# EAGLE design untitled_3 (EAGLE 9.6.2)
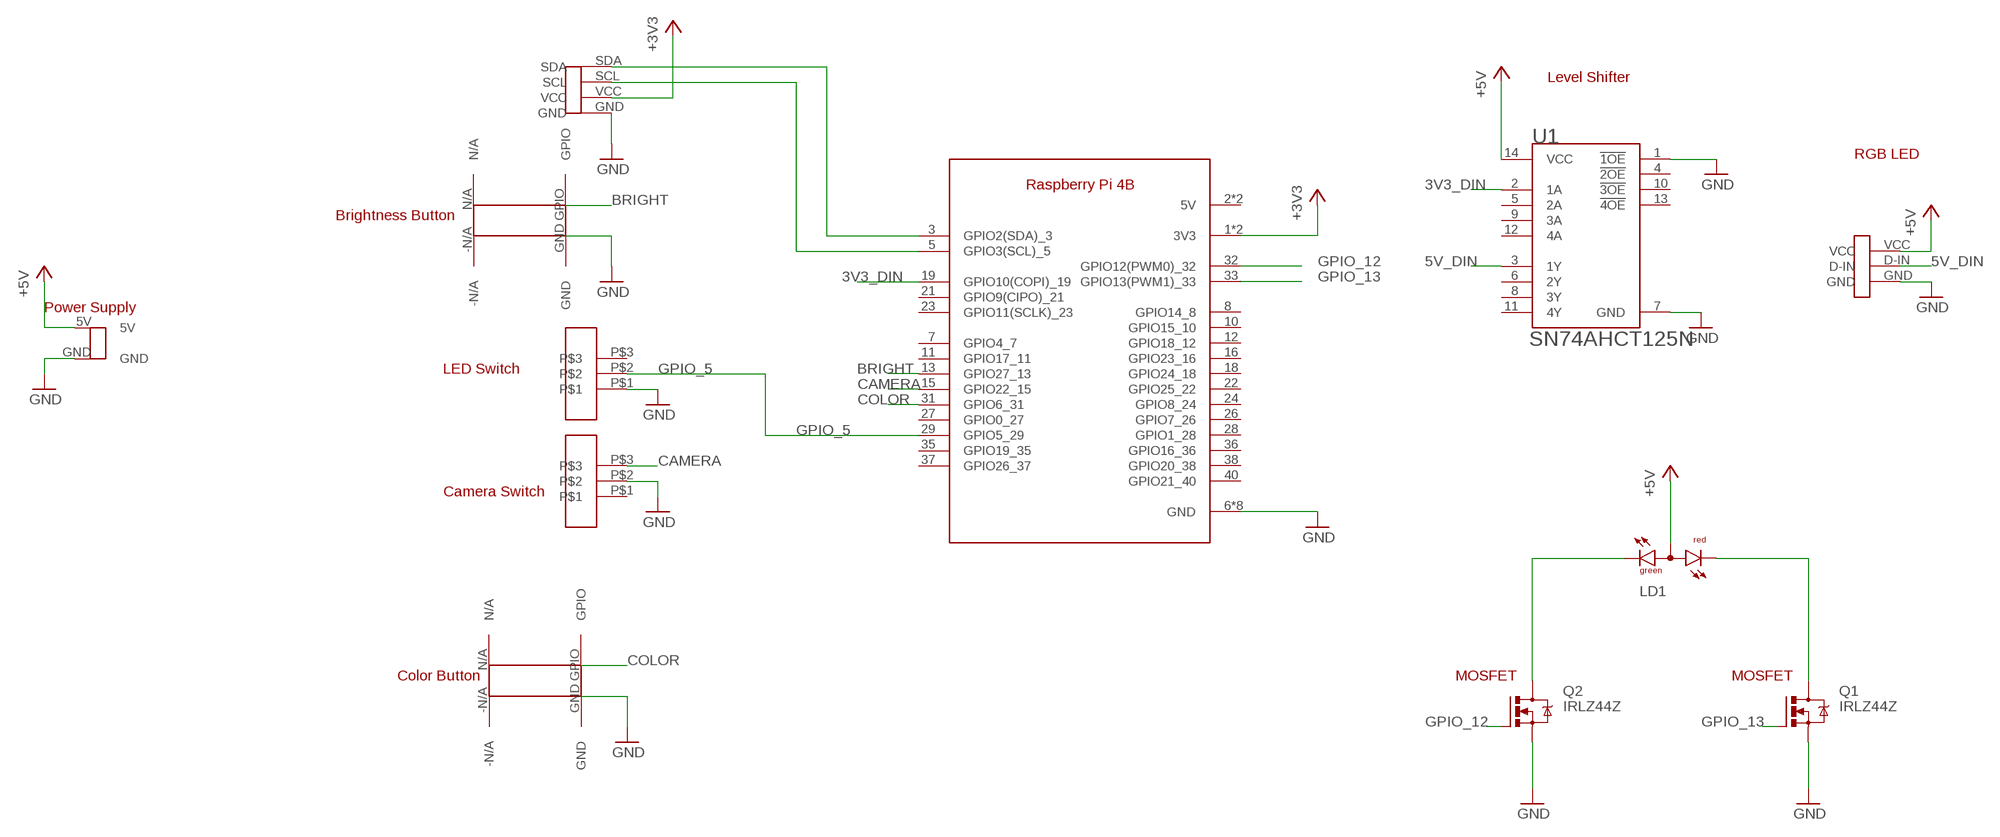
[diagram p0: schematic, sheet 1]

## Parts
LD1  DUOLED-RG-A  [DUOLED-A-5MM]
Q1  IRLZ44Z  [TO220BH]
Q2  IRLZ44Z  [TO220BH]
U1  TEXAS_INSTRUMENTS_SN74AHCT125NTEXAS_INSTRUMENTS_SN74AHCT125N_0_0  [TEXAS_INSTRUMENTS_SN74AHCT125N_0]
U$1  RASPBERRY_PI_4  [RASPI_4B]
U$2  G13-SW  [G13-SW]
U$3  G13-SW  [G13-SW]
U$4  LIGHTSENSOR-PO  [LIGHTSENSOR-IO]
U$5  LED-STRIP-PO  [LED-STRIP-PO]
U$6  G13-BUTTON  [G13-BUTTON]
U$7  G13-BUTTON  [G13-BUTTON]
U$8  G13-BATTERY  [G13-BATTERY]

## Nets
3V3_DIN: U1.2(1A) U$1.19(GPIO10(COPI)_19)
5V_DIN: U1.3(1Y) U$5.D-IN
+3V3: U$1.1(3V3) U$1.17(3V3) U$4.VCC
+5V: LD1.A U1.14(VCC) U$5.VCC U$8.5V
BRIGHT: U$1.13(GPIO27_13) U$6.GPIO
CAMERA: U$1.15(GPIO22_15) U$3.P$3
COLOR: U$1.31(GPIO6_31) U$7.GPIO
GND: Q1.S Q2.S U1.1(!1OE!) U1.7(GND) U$1.6(GND) U$1.9(GND) U$1.14(GND) U$1.20(GND) U$1.25(GND) U$1.30(GND) U$1.34(GND) U$1.39(GND) U$2.P$1 U$3.P$2 U$4.GND U$5.GND U$6.GND U$7.GND U$8.GND
GPIO_5: U$1.29(GPIO5_29) U$2.P$2
GPIO_12: Q2.G U$1.32(GPIO12(PWM0)_32)
GPIO_13: Q1.G U$1.33(GPIO13(PWM1)_33)
N$1: U$1.3(GPIO2(SDA)_3) U$4.SDA
N$2: U$1.5(GPIO3(SCL)_5) U$4.SCL
N$3: LD1.CR Q1.D
N$12: LD1.CX(CG) Q2.D
Unconnected: U1.4(!2OE!) U1.5(2A) U1.6(2Y) U1.8(3Y) U1.9(3A) U1.10(!3OE!) U1.11(4Y) U1.12(4A) U1.13(!4OE!) U$1.2(5V) U$1.4(5V) U$1.7(GPIO4_7) U$1.8(GPIO14_8) U$1.10(GPIO15_10) U$1.11(GPIO17_11) U$1.12(GPIO18_12) U$1.16(GPIO23_16) U$1.18(GPIO24_18) U$1.21(GPIO9(CIPO)_21) U$1.22(GPIO25_22) U$1.23(GPIO11(SCLK)_23) U$1.24(GPIO8_24) U$1.26(GPIO7_26) U$1.27(GPIO0_27) U$1.28(GPIO1_28) U$1.35(GPIO19_35) U$1.36(GPIO16_36) U$1.37(GPIO26_37) U$1.38(GPIO20_38) U$1.40(GPIO21_40) U$2.P$3 U$3.P$1 U$6.-N/A U$6.N/A U$7.-N/A U$7.N/A

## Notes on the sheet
- Level Shifter
- RGB LED
- Brightness Button
- Power Supply
- LED Switch
- Camera Switch
- Color Button | MOSFET | MOSFET

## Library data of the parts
LD1 = led:DUOLED-RG-A: DUO LED 2 colors (red/green), 5 mm, round, common Anode www.ligitek.com or other producers.
Q1 Q2 = transistor-power:IRLZ44Z: N-Channel HEXFET® Power MOSFET Logic Level AUTOMOTIVE MOSFET Source: http://www.irf.com/product-info/datasheets/data/irlz44zpbf.pdf
U1 = Texas Instruments - SN74AHCT125N:TEXAS_INSTRUMENTS_SN74AHCT125N: QUADRUPLE BUS BUFFER GATES WITH 3-STATE OUTPUTS; CENTROID_NOT_SPECIFIED: No; DATASHEET: http://www.ti.com/lit/ds/symlink/sn74ahct125.pdf; DIGIKEY_DESCRIPTION: IC BUS BUFFER TRI-ST QD 14DIP; DIGIKEY_PART_NUMBER: 296-4655-5-ND; IPC_LAND_PATTERN_NAME: DIP794W46P254L1930H508Q14; LEAD_FREE: yes; MF: Texas Instruments; MOUSER_PART_NUMBER: 595-SN74AHCT125N; MPN: SN74AHCT125N; PACKAGE: PDIP-14; PREFIX: U; ROHS: yes; TEMPERATURE_RANGE_HIGH: +125°C; TEMPERATURE_RANGE_LOW: -40°C
U$1 = raspberryPi4:RASPBERRY_PI_4
U$2 U$3 = raspberryPi4:G13-SW
U$4 = raspberryPi4:LIGHTSENSOR-PO
U$5 = raspberryPi4:LED-STRIP-PO
U$6 U$7 = sumayyah:G13-BUTTON
U$8 = raspberryPi4:G13-BATTERY

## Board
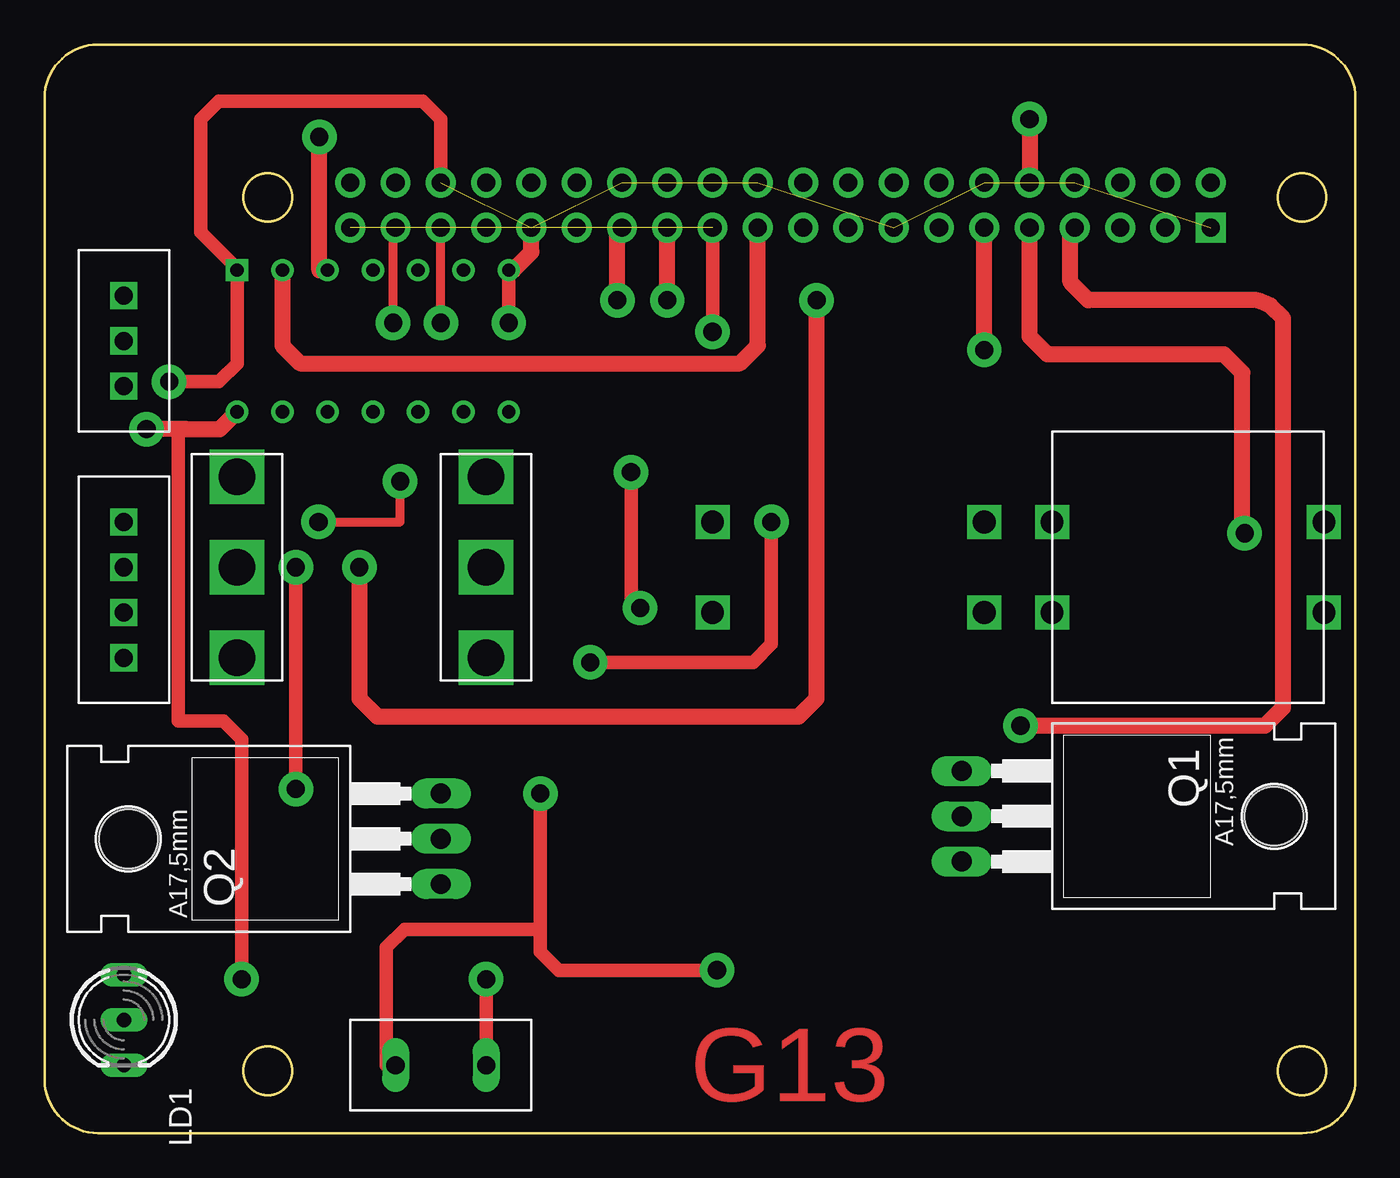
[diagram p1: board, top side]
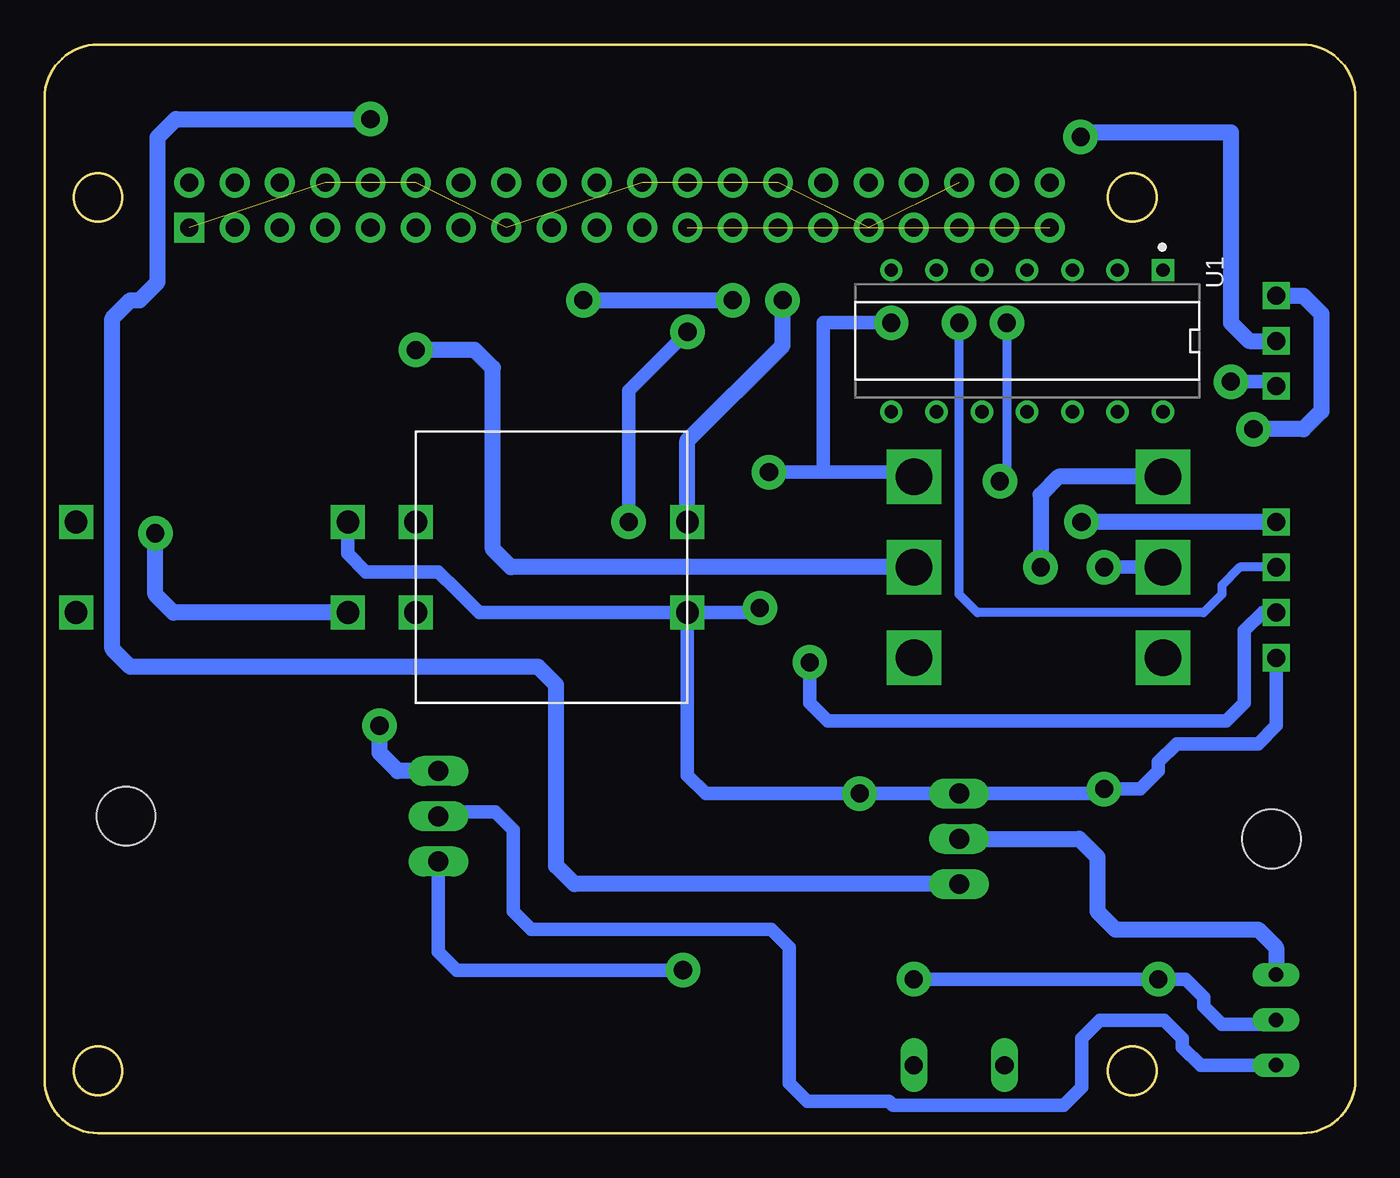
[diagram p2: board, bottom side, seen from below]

Size 73.52 x 61.08 mm. Coordinates in mm from the lower left corner, seen from the top.
Outline: 73.52,3 73.52,58.08 arc90 70.53,61.08 3,61.08 arc90 0,58.08 0,3 arc90 3,0 70.52,0 arc90 73.52,3
Outline: circle at 70.52,52.5 radius 1.35
Outline: circle at 70.52,3.5 radius 1.35
Outline: circle at 12.53,52.5 radius 1.35
Outline: circle at 12.53,3.5 radius 1.35
Copper layers (1*16): Top 0.035mm / dielectric 1.5mm / Bottom 0.035mm
Design rules "default": minimum track width 6mil, minimum drill 0.35mm, track to track 6mil, track to pad 6mil, pad to pad 6mil, via to via 6mil, smd to smd 6mil, copper to edge 40mil, drill to drill 6mil, minimum pad ring 10mil, minimum via ring 8mil, stop-mask expansion 4mil, vias tented up to drill 0mil, thermal gap 10mil

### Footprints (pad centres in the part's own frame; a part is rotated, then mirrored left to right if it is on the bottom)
DUOLED-A-5MM = drill 0.813 long: A 0,0; CR 2.54,0; CX -2.54,0
TO220BH = drill 1.118 long: D 0,-6.35; G -2.54,-6.35; S 2.54,-6.35 | hole 3.302: 0,11.176
TEXAS_INSTRUMENTS_SN74AHCT125N_0 = drill 0.75 pad 1.25 square: 1 -3.97,7.62 | drill 0.75 pad 1.25: 2 -3.97,5.08; 3 -3.97,2.54; 4 -3.97,0; 5 -3.97,-2.54; 6 -3.97,-5.08; 7 -3.97,-7.62; 8 3.97,-7.62; 9 3.97,-5.08; 10 3.97,-2.54; 11 3.97,0; 12 3.97,2.54; 13 3.97,5.08; 14 3.97,7.62
RASPI_4B = drill 1.016 pad 1.676: 1 -24.13,-1.27; 2 -24.13,1.27; 3 -21.59,-1.27; 4 -21.59,1.27; 5 -19.05,-1.27; 6 -19.05,1.27; 7 -16.51,-1.27; 8 -16.51,1.27; 9 -13.97,-1.27; 10 -13.97,1.27; 11 -11.43,-1.27; 12 -11.43,1.27; 13 -8.89,-1.27; 14 -8.89,1.27; 15 -6.35,-1.27; 16 -6.35,1.27; 17 -3.81,-1.27; 18 -3.81,1.27; 19 -1.27,-1.27; 20 -1.27,1.27; 21 1.27,-1.27; 22 1.27,1.27; 23 3.81,-1.27; 24 3.81,1.27; 25 6.35,-1.27; 26 6.35,1.27; 27 8.89,-1.27; 28 8.89,1.27; 29 11.43,-1.27; 30 11.43,1.27; 31 13.97,-1.27; 32 13.97,1.27; 33 16.51,-1.27; 34 16.51,1.27; 35 19.05,-1.27; 36 19.05,1.27; 37 21.59,-1.27; 38 21.59,1.27; 40 24.13,1.27 | drill 1.016 pad 1.676 square: 39 24.13,-1.27
G13-SW = drill 2.032 square: P$1 -5.08,0; P$2 0,0; P$3 5.08,0
LIGHTSENSOR-IO = drill 1.016 square: GND -5.08,0; SCL 0,0; SDA 2.54,0; VCC -2.54,0
LED-STRIP-PO = drill 1.016 square: D-IN 0,0; GND -2.54,0; VCC 2.54,0
G13-BUTTON = drill 1.27 square: -N/A -7.62,-2.54; GND 7.62,-2.54; GPIO 7.62,2.54; N/A -7.62,2.54
G13-BATTERY = drill 1.016 long: 5V -2.54,0; GND 2.54,0

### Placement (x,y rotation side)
LD1  4.45,6.35 270 top
Q1  57.79,17.78 270 top
Q2  15.88,16.51 90 top
U1  18.41,44.45 270 bottom
U$1  41.27,52.07 0 top
U$2  24.76,31.75 270 top
U$3  10.79,31.75 90 top
U$4  4.45,31.75 90 top
U$5  4.45,44.45 90 top
U$6  45.09,31.75 0 bottom
U$7  64.13,31.75 180 top
U$8  22.22,3.81 180 top

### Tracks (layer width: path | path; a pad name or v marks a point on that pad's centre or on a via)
3V3_DIN
  Top 0.889: U1.2 13.34,44.2 14.35,43.18 38.99,43.18 40.01,44.2 U$1.19
5V_DIN  (via drill 1.02 pad 1.93)
  Top 0.889: U1.3 15.41,48.42 v15.41,55.9
  Bottom 0.889: v15.41,55.9 15.16,56.15 6.99,56.15 6.99,45.47 5.97,44.45 U$5.D-IN
+3V3  (via drill 1.02 pad 1.93)  (1 unrouted)
  Top 0.762: U$1.17 v37.47,44.96 | v40.77,34.29 40.77,27.43 39.75,26.42 v30.61,26.42
  Bottom 0.762: v37.47,44.96 40.77,41.66 v40.77,34.29 | v30.61,26.42 30.61,24.13 29.59,23.11 7.24,23.11 6.22,24.13 6.22,28.19 5.21,29.21 U$4.VCC
+5V  (via drill 1.02 pad 1.93)
  Top 0.762: U$8.5V v24.76,8.64 | v11.05,8.64 11.05,22.1 10.03,23.11 7.49,23.11 7.49,39.5 8,39.5
  Top 0.889: U1.14 9.81,39.5 8,39.5 v5.71,39.5
  Bottom 0.762: v24.76,8.64 v11.05,8.64 9.53,8.64 8.51,7.62 8.51,7.11 7.49,6.1 4.45,6.1 LD1.A
  Bottom 0.889: U$5.VCC 2.92,46.99 1.91,45.97 1.91,40.51 2.92,39.5 v5.71,39.5
BRIGHT  (via drill 1.02 pad 1.93)
  Top 0.889: v32.13,46.74 32.13,50.8 U$1.13
  Bottom 0.889: U$6.GPIO 37.47,38.86 32.13,44.2 v32.13,46.74
CAMERA  (via drill 1.02 pad 1.93)
  Top 0.889: v17.65,31.75 17.65,24.38 18.67,23.37 42.29,23.37 43.31,24.38 v43.31,46.74 | v34.93,46.74 U$1.15
  Bottom 0.889: U$3.P$3 16.64,36.83 17.65,35.81 v17.65,31.75 | v43.31,46.74 v34.93,46.74
COLOR  (via drill 1.02 pad 1.93)
  Top 0.889: v67.31,33.66 67.18,33.66 67.18,42.67 66.17,43.69 56.26,43.69 55.25,44.7 U$1.31
  Bottom 0.889: U$7.GPIO 66.29,29.21 67.31,30.23 v67.31,33.66
GND  (via drill 1.02 pad 1.93)  (7 unrouted)
  Top 0.762: U$8.GND 19.18,3.81 19.18,10.41 20.19,11.43 27.81,11.43 | 27.81,11.43 v27.81,19.05 | v33.4,29.46 32.89,29.46 v32.89,37.08 | U1.7 v26.04,45.47 | v37.72,9.14 28.83,9.14 27.81,10.16 27.81,11.43 | v6.99,42.16 9.78,42.16 10.79,43.18 U1.1 10.79,48.51 9.78,49.53 8.76,50.55 8.76,56.9 9.78,57.91 21.21,57.91 22.22,56.9 U$1.6 | v14.1,19.3 v14.1,31.75
  Top 0.889: U1.7 26.29,48.42 27.3,49.44 U$1.9
  Bottom 0.762: U$6.GND 37.47,20.07 36.45,19.05 v27.81,19.05 Q2.S 14.1,19.05 v14.1,19.3 12.06,19.3 11.05,20.32 11.05,20.83 10.03,21.84 5.46,21.84 4.45,22.86 U$4.GND | U$6.GND 33.4,29.21 v33.4,29.46 | v32.89,37.08 29.84,37.08 | 29.84,37.08 24.76,37.08 U$2.P$1 | 29.84,37.08 29.84,45.47 v26.04,45.47 | Q1.S 51.44,10.16 50.42,9.14 v37.72,9.14 | U$7.GND 56.52,32.51 55.5,31.5 51.44,31.5 50.42,30.48 49.15,29.21 U$6.GND | U$5.GND 4.45,42.16 v6.99,42.16 | v14.1,31.75 U$3.P$2
GPIO_5  (via drill 1.02 pad 1.93)
  Top 0.889: v52.71,43.94 U$1.29
  Bottom 0.889: U$2.P$2 47.37,31.75 48.39,32.77 48.39,42.93 49.4,43.94 v52.71,43.94
GPIO_12  (via drill 1.02 pad 1.93)
  Top 0.889: v55.25,56.9 U$1.32
  Bottom 0.889: Q2.G 43.82,13.97 44.83,14.99 44.83,25.15 45.85,26.16 68.71,26.16 69.72,27.18 69.72,45.72 68.71,46.74 68.2,46.74 67.18,47.75 67.18,55.88 66.17,56.9 v55.25,56.9
GPIO_13  (via drill 1.02 pad 1.93)
  Top 0.889: v54.74,22.86 68.45,22.86 69.47,23.88 69.47,45.72 68.75,46.44 68.03,46.74 58.55,46.74 57.53,47.75 57.53,50.8 U$1.33
  Bottom 0.889: Q1.G 53.72,20.32 54.74,21.34 v54.74,22.86
N$1  (via drill 1.02 pad 1.93)
  Top 0.508: v15.37,34.29 19.94,34.29 v19.94,36.58 | v19.55,45.47 19.55,50.8 U$1.3
  Bottom 0.508: v19.55,45.47 19.55,36.96 v19.94,36.58
  Bottom 0.889: U$4.SDA v15.37,34.29
N$2  (via drill 1.02 pad 1.93)
  Top 0.508: v22.22,45.47 U$1.5
  Bottom 0.508: U$4.SCL 6.48,31.75 7.49,30.73 7.49,30.23 8.51,29.21 21.21,29.21 22.22,30.23 v22.22,45.47
N$3
  Bottom 0.762: LD1.CR 8.69,3.81 9.7,4.83 9.7,5.31 10.72,6.32 14.33,6.32 15.35,5.31 15.35,2.56 16.36,1.55 25.93,1.55 26.16,1.78 30.73,1.78 31.75,2.79 31.75,10.41 32.77,11.43 46.23,11.43 47.24,12.45 47.24,17.02 48.26,18.03 51.44,18.03 Q1.D
N$12
  Bottom 0.889: Q2.D 15.49,16.51 14.48,15.49 14.48,12.45 13.46,11.43 5.46,11.43 4.45,10.41 LD1.CX

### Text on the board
Top: G13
